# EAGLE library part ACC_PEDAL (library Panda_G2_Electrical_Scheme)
Accelerator pedal
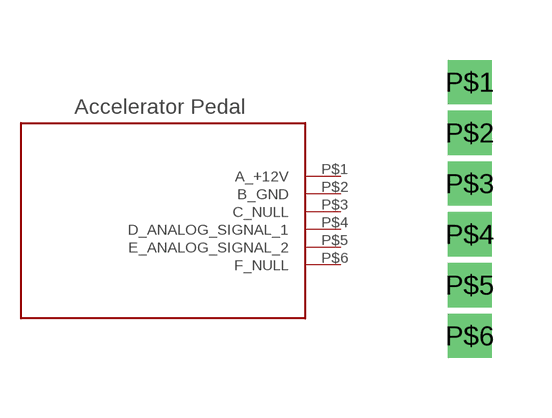
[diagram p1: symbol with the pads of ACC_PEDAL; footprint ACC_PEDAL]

Designator prefix -

## ACC_PEDAL  [ACC_PEDAL]
P$1  A_+12V
P$2  B_GND
P$3  C_NULL
P$4  D_ANALOG_SIGNAL_1
P$5  E_ANALOG_SIGNAL_2
P$6  F_NULL

## Footprint ACC_PEDAL (pad centres in mm)
drill 0.6 square: P$1 5.08,11.43; P$2 5.08,10.16; P$3 5.08,8.89; P$4 5.08,7.62; P$5 5.08,6.35; P$6 5.08,5.08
